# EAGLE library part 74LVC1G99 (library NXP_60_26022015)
Ultra-configurable multiple function gate; 3-state The 74LVC1G99 provides a low voltage, ultra-configurable, multiple function gate with 3-state output. The device can be configured as one of several logic functions including, AND, OR, NAND, NOR, XOR, XNOR, inverter, buffer and MUX. No external components are required to configure the device as all inputs can be connected directly to VCC or GND. The 3-state output is controlled by the output enable input (OE). A HIGH level at OE causes the output (Y) to assume a high-impedance OFF-state. When OE is LOW, the output state is determined by the signals applied to the Schmitt trigger inputs (A, B, C and D). Due to the use of Schmitt trigger inputs the device is tolerant of slowly changing input signals, transforming them into sharply defined, jitter free output signals. By eliminating leakage current paths to VCC and GND, the inputs and disabled output are also over-voltage tolerant, making the device suitable for mixed-voltage applications. This device is fully specified for partial power-down applications using IOFF. The IOFF circuitry disables the output, preventing the damaging backflow current through the device when it is powered down. The 74LVC1G99 is fully specified over the supply range from 1.65 V to 5.5 V. AAL Eindhoven MK
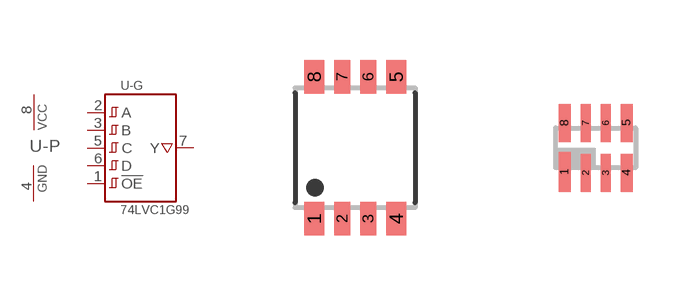
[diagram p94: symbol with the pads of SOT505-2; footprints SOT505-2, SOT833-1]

Designator prefix U; gates -G=74LVC1G99 -P=PWRN

## 74LVC1G99DP  [SOT505-2]
1  -G:!OE!  in
2  -G:A  in
3  -G:B  in
4  -P:GND  pwr
5  -G:C  in
6  -G:D  in
7  -G:Y  out
8  -P:VCC  pwr

## 74LVC1G99GT  [SOT833-1]
Pads as for SOT505-2

## 74LVC1G99GF  [SOT1089-1]
Pads as for SOT505-2

## 74LVC1G99GD  [SOT996-2/3]
Pads as for SOT505-2

## 74LVC1G99GM  [SOT902-1/2/3]
1  -G:Y  out
2  -G:D  in
3  -G:C  in
4  -P:GND  pwr
5  -G:B  in
6  -G:A  in
7  -G:!OE!  in
8  -P:VCC  pwr

## 74LVC1G99GS  [SOT1203]
Pads as for SOT505-2

## Footprint SOT505-2 (pad centres in mm)
SOT505-2 TSSOP8: plastic thin shrink small outline package; 8 leads; body width 3 mm JEDEC: -- IEC: --
smd 0.5 x 0.85: 1 -1.025,-1.775; 4 1.025,-1.775; 5 1.025,1.775; 8 -1.025,1.775
smd 0.4 x 0.85: 2 -0.325,-1.775; 3 0.325,-1.775; 6 0.325,1.775; 7 -0.325,1.775

## Footprint SOT833-1 (pad centres in mm)
SOT833-1 XSON8: plastic extremely thin small outline package; no leads; 8 terminals; body 1 x 1.95 x 0.5 mm JEDEC: MO-252 IEC: -- JEITA: --
smd 0.3 x 1: 1 -0.775,-0.6
smd 0.25 x 0.95: 2 -0.25,-0.625; 3 0.25,-0.625; 6 0.25,0.625; 7 -0.25,0.625
smd 0.3 x 0.95: 4 0.775,-0.625; 5 0.775,0.625; 8 -0.775,0.625

## Footprint SOT1089-1 (pad centres in mm)
SOT1089-1 XSON8: plastic, extremely thin small outline package; no leads; 8 terminals; body 1 x 1.35 x 0.5 mm JEDEC: -- IEC: -- JEITA: --
smd 0.15 x 0.5: 1 -0.525,-0.35; 2 -0.175,-0.35; 3 0.175,-0.35; 4 0.525,-0.35; 5 0.525,0.35; 6 0.175,0.35; 7 -0.175,0.35; 8 -0.525,0.35

## Footprint SOT996-2/3 (pad centres in mm)
SOT996-2/3 XSON8U: plastic extremely thin small outline package; no leads;8 terminals; UTLP based; body 3 x 2 x 0.5 mm JEDEC: IEC: -- JEITA: --
smd 0.25 x 1.1: 1 -0.75,-1.45
smd 0.25 x 1: 2 -0.25,-1.5; 3 0.25,-1.5; 4 0.75,-1.5; 5 0.75,1.5; 6 0.25,1.5; 7 -0.25,1.5; 8 -0.75,1.5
